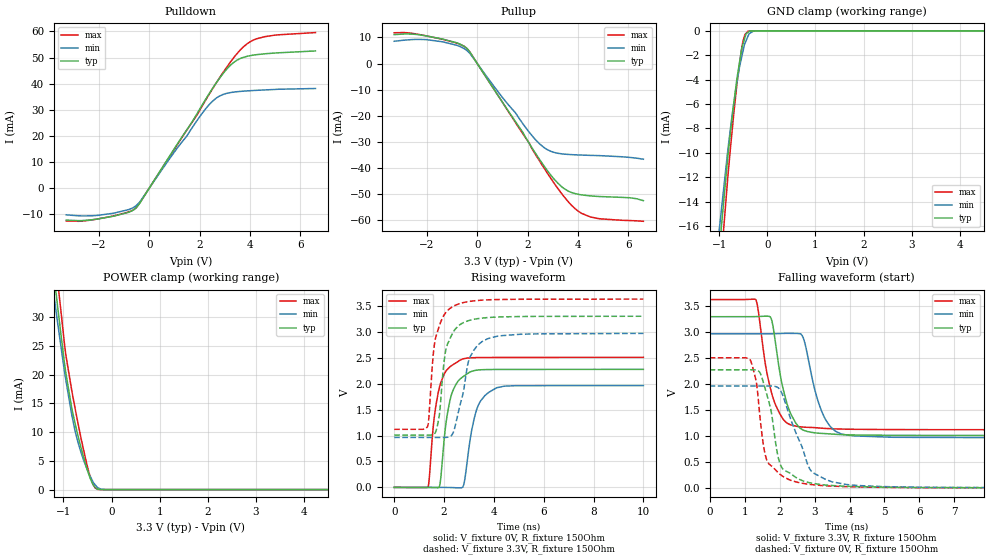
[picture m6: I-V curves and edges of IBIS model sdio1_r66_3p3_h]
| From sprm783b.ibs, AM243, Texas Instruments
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|   r66_3p3_h
[Model]   sdio1_r66_3p3_h
Model_type   I/O
Polarity   Non-Inverting
Enable   Active-High
Vinl = 0
Vinh = 0.8
Vmeas = 1.65
Vref = 3.3
Cref = 2pF
Rref = 100000
|   typ   min   max
C_comp   5.631pF   5.516pF   5.647pF
[Voltage Range]   3.3   2.97   3.63
[Temperature Range]   27   150   -40
[Pullup Reference]   3.3   2.97   3.63
[Pulldown Reference]   0   0   0
[Power Clamp Reference]   3.3   2.97   3.63
[GND Clamp Reference]   0   0   0
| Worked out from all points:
|   slope of the pulldown table from 0 to 0.495 V, typ, clamps not added: 65.6 ohm
|   slope of the pullup table from 0 to 0.495 V, typ, clamps not added: 67.1 ohm
|   GND clamp passes 1 mA (typ) near -0.50 V on its own axis
|   POWER clamp passes 1 mA (typ) near -0.39 V on its own axis
|   falling waveform, V_fixture 3.3V, R_fixture 150Ohm: 20-80 % time 422ps typ, 482ps min, 425ps max; typ from 3.3 V to 1.01 V
|   rising waveform, V_fixture 0V, R_fixture 150Ohm: 20-80 % time 400ps typ, 463ps min, 402ps max; typ from 0.001 V to 2.28 V
|   rising waveform, V_fixture 3.3V, R_fixture 150Ohm: 20-80 % time 387ps typ, 572ps min, 392ps max; typ from 1.01 V to 3.3 V
|   falling waveform, V_fixture 0V, R_fixture 150Ohm: 20-80 % time 392ps typ, 646ps min, 317ps max; typ from 2.28 V to 0.001 V
[Pulldown]
|   Voltage   I(typ)   I(min)   I(max)
-3.3V     -12.31mA   -10.29mA   -12.62mA
-2.043V   -11.85mA   -10.47mA   -11.85mA
-825mV    -9.307mA   -8.287mA   -9.206mA
-528mV    -7.654mA   -6.783mA   -7.589mA
1.907V    28.69mA    26.04mA    28.23mA
2.363V    35.95mA    31.79mA    35.7mA
2.779V    41.93mA    35.18mA    42.05mA
3.194V    46.78mA    36.52mA    47.91mA
3.462V    48.86mA    36.88mA    51.25mA
3.887V    50.48mA    37.21mA    55.29mA
4.274V    51.11mA    37.44mA    57.21mA
6.6V      52.52mA    38.13mA    59.57mA
[GND Clamp]
|   Voltage   I(typ)   I(min)   I(max)
-3.3V     -160mA     -119.4mA   -217mA
-1.013V   -18.47mA   -16.75mA   -21.37mA
-825mV    -10.43mA   -9.89mA    -12.11mA
-716.1mV  -6.532mA   -6.434mA   -7.501mA
-627mV    -3.775mA   -4.073mA   -4.142mA
-537.9mV  -1.565mA   -2.22mA    -1.565mA
-508.2mV  -1.103mA   -1.688mA   -876.2uA
-448.8mV  -317.7uA   -866.7uA   -227.1uA
-399.3mV  -111.5uA   -410.6uA   -25.47uA
-300.3mV  -2.826uA   -47.28uA   -741.7nA
-132mV    -44.77nA   -1.775uA   -83.62nA
6.6V      0A         0A         0A
[Pullup]
|   Voltage   I(typ)   I(min)   I(max)
-3.3V     11.09mA    8.547mA    11.81mA
-2.033V   10.62mA    9.184mA    10.64mA
-825mV    7.986mA    7.034mA    7.893mA
-409.2mV  5.742mA    4.952mA    5.767mA
2.056V    -30.5mA    -26.26mA   -30.44mA
2.363V    -35.19mA   -29.75mA   -35.68mA
2.917V    -42.78mA   -33.67mA   -44.01mA
3.472V    -48.14mA   -34.78mA   -51.39mA
4.026V    -50.23mA   -35.1mA    -56.77mA
4.491V    -50.81mA   -35.25mA   -58.87mA
6.056V    -51.52mA   -36.03mA   -60.27mA
6.6V      -52.64mA   -36.73mA   -60.56mA
[POWER Clamp]
|   Voltage   I(typ)   I(min)   I(max)
-3.3V     224.5mA    191.3mA    262.6mA
-1.191V   37.07mA    33.44mA    42.47mA
-1.132V   32.63mA    29.7mA     37.31mA
-1.122V   31.9mA     29.08mA    36.46mA
-953.7mV  20.48mA    19.24mA    23.62mA
-825mV    14.08mA    12.93mA    17.14mA
-765.6mV  11.79mA    10.51mA    14.49mA
-627mV    7.039mA    6.292mA    8.648mA
-468.6mV  2.565mA    2.728mA    2.954mA
-399.3mV  1.162mA    1.563mA    1.166mA
-290.4mV  108.6uA    361.9uA    43.24uA
6.6V      0A         0A         0A
[Ramp]
R_load = 150
|   typ   min   max
dV/dt_r   1.36524/3.98873e-10   1.17722/4.62538e-10   1.50402/4.01319e-10
dV/dt_f   1.37491/4.21688e-10   1.20325/4.81427e-10   1.50573/4.25408e-10
[Falling Waveform]
V_fixture = 3.3V
V_fixture_min = 2.97V
V_fixture_max = 3.63V
R_fixture = 150Ohm
C_fixture = 0F
|   Time   V(typ)   V(min)   V(max)
0s        3.3V       2.969V     3.63V
1.325ns   3.302V     2.969V     3.623V
1.6ns     3.309V     2.969V     2.359V
1.735ns   3.295V     2.97V      1.929V
2.06ns    2.033V     2.976V     1.367V
2.31ns    1.443V     2.978V     1.218V
2.65ns    1.123V     2.931V     1.173V
3.19ns    1.051V     1.499V     1.151V
3.76ns    1.027V     1.041V     1.134V
10ns      1.008V     963.6mV    1.12V
[Rising Waveform]
V_fixture = 0V
V_fixture_min = 0V
V_fixture_max = 0V
R_fixture = 150Ohm
C_fixture = 0F
|   Time   V(typ)   V(min)   V(max)
0s        610.1uV    1.364mV    475.9uV
1.36ns    317.2uV    852uV      8.857mV
1.595ns   -2.069mV   655.3uV    1.3V
1.805ns   3.817mV    647.5uV    1.91V
2.225ns   1.648V     -1.559mV   2.318V
2.66ns    2.096V     -7.904mV   2.457V
2.815ns   2.151V     104.6mV    2.484V
3.325ns   2.262V     1.523V     2.503V
4.105ns   2.274V     1.92V      2.505V
10ns      2.276V     1.963V     2.507V
[Rising Waveform]
V_fixture = 3.3V
V_fixture_min = 2.97V
V_fixture_max = 3.63V
R_fixture = 150Ohm
C_fixture = 0F
|   Time   V(typ)   V(min)   V(max)
0s        1.008V     963.6mV    1.12V
1.335ns   1.008V     963.4mV    1.17V
1.555ns   1.017V     963.2mV    2.493V
1.645ns   1.052V     963.2mV    2.848V
1.815ns   1.404V     963.2mV    3.119V
2.06ns    2.62V      964.1mV    3.365V
2.4ns     3.019V     1.099V     3.499V
3.03ns    3.222V     2.5V       3.586V
3.735ns   3.274V     2.862V     3.615V
10ns      3.3V       2.969V     3.63V
[Falling Waveform]
|Gnd
V_fixture = 0V
V_fixture_min = 0V
V_fixture_max = 0V
R_fixture = 150Ohm
C_fixture = 0F
|   Time   V(typ)   V(min)   V(max)
0s        2.276V     1.963V     2.507V
1.16ns    2.276V     1.964V     2.464V
1.34ns    2.27V      1.964V     2.017V
1.42ns    2.238V     1.964V     1.5V
1.645ns   1.777V     1.964V     518.2mV
1.99ns    512.2mV    1.912V     275mV
2.31ns    277.3mV    1.341V     148.5mV
2.87ns    97.54mV    357.4mV    66.65mV
3.51ns    44.83mV    115.4mV    33.36mV
10ns      618.8uV    1.365mV    475.9uV
